| IBIS file stm32u5f9_5g9_ufbga144_dsi_smps.ibs
[IBIS ver] 4.2
[File name] stm32u5f9_5g9_ufbga144_dsi_smps.ibs
[File Rev] 1.0
[Date]  29-10-2024
[Source] Data Created at STMicroelectronics
[Notes]  File originated from ELDO simulations.
[Disclaimer]  This information is for modeling purpose only and is
   not guaranteed. The information is subject to change without
   notice.
[Copyright] Copyright 2024 STMicroelectronics Inc.
|   Component stm32u5f9_5g9_ufbga144_dsi_smps
[Component] stm32u5f9_5g9_ufbga144_dsi_smps
[Manufacturer] STMicroelectronics
[Package]
| variable   typ   min   max
R_pkg  0  NA  NA
L_pkg  0  NA  NA
C_pkg  0  NA  NA
[Pin]   signal_name   model_name
A1  VSS  gnd
A2  PB9  io8_100m_hslv_ft
A3  PH3-BOOT0  io8_100m_ft
A4  PB6  io8_100m_i2c_ft
A5  PB4  io8_100m_hslv_ft
A6  PG14  io8_100m_hslv_ft
A7  PG12  io8_100m_hslv_ft
A8  PG10  io8_100m_hslv_ft
A9  PD7  io8_100m_hslv_ft
A10  PD3  io8_166m_hslv_ft
A11  PC12  io8_166m_hslv_ft
A12  VSS  gnd
B1  PE2  io8_100m_hslv_ft
B2  PE3  io8_100m_hslv_tamp_ft
B3  PE0  io8_100m_hslv_ft
B4  PB8  io8_100m_hslv_ft
B5  PB5  io8_166m_hslv_ft
B6  PG15  io8_100m_hslv_ft
B7  PG9  io8_100m_hslv_ft
B8  PD5  io8_100m_hslv_ft
B9  PD2  io8_100m_hslv_ft
B10  PC10  io8_100m_hslv_ft
B11  PA14  io8_100m_ft
B12  PA10  io8_100m_usb_id
C1  PC14-OSC32_IN   io8_100m_ft
C2  VBAT  power
C3  PE4  io8_100m_hslv_tamp_ft
C4  PE5  io8_100m_hslv_tamp_ft
C5  PB7  io8_166m_hslv_i2c_ft
C6  PG13  io8_100m_hslv_ft
C7  PD4  io8_100m_hslv_ft
C8  PC11  io8_100m_hslv_ft
C9  PA15  nc
C10  PA13  io8_100m_ft
C11  PA12  io8_100m_ft
C12  PA11  io8_100m_ft
D1  VSSDSI  nc
D2  PC15-OSC32_OUT  io8_100m_ft
D3  PE6  io8_100m_hslv_tamp_ft
D4  VDD11  nc
D5  VSS  gnd
D6  PB3  io8_100m_hslv_ft
D7  PD6  io8_166m_hslv_ft
D8  PD0  io8_100m_hslv_ft
D9  VSS  gnd
D10  VDDUSB  power
D11  PA8  io8_166m_hslv_ft
D12  PC8  io8_100m_hslv_ft
E1  DSI_D0N  nc
E2  DSI_D0P  nc
E3  VDDDSI  nc
E4  PC13  io8_100m_ft_v33
E5  PF0  io8_100m_hslv_ft
E6  VDDIO2  power
E7  PD1  io8_100m_hslv_ft
E8  VDD  power
E9  PA9  io8_100m_usb_vbus_ft
E10  VDD  power
E11  PI2  io8_spi_ft
E12  PI3  io8_spi_ft
F1  DSI_CKN  nc
F2  DSI_CKP  nc
F3  VSSDSI  nc
F4  PF1  io8_100m_hslv_ft
F5  VDD  power
F6  VSS  gnd
F7  VSS  gnd
F8  PC9  io8_100m_hslv_ft
F9  PC7  io8_100m_hslv_ft
F10  VSS  gnd
F11  PI0  io8_spi_ft
F12  PI1  io8_spi_ft
G1  DSI_D1N  nc
G2  DSI_D1P  nc
G3  VDD11DSI  nc
G4  PF2  io8_100m_hslv_ft
G5  PC2  io8_100m_hslv_ft
G6  VSS  gnd
G7  VSS  gnd
G8  VDD  power
G9  PC6  io8_100m_hslv_ft
G10  VDD  power
G11  PH14  io8_spi_ft
G12  PH15  io8_spi_ft
H1  VSSDSI  nc
H2  PH0-OSC_IN  io8_100m_ft
H3  VREFP  nc
H4  PA0  io8_100m_hslv_tamp_ft
H5  VDD  power
H6  PB2  io8_100m_hslv_tamp_ft
H7  VDD  power
H8  PE8  io8_100m_hslv_ft
H9  PD15  io8_100m_hslv_ft
H10  VSS  gnd
H11  PH12  io8_spi_ft
H12  PH13  io8_spi_ft
J1  PH1-OSC_OUT  io8_100m_ft
J2  NRST  nc
J3  VSSA  nc
J4  VDDA  nc
J5  PB0  io8_100m_hslv_ft
J6  PG1  io8_100m_hslv_ft
J7  PE10  io8_166m_hslv_ft
J8  PE12  io8_100m_hslv_ft
J9  VDD11  nc
J10  VDD  power
J11  PH11  io8_spi_ft
J12  PH10  io8_spi_ft
K1  PC1  io8_166m_hslv_i2c_ft
K2  PC0  io8_100m_hslv_ft
K3  PA1  io8_100m_hslv_tamp_ft
K4  PA5  io8_100m_ft
K5  PG0  io8_100m_hslv_ft
K6  PE9  io8_166m_hslv_ft
K7  PE14  io8_100m_hslv_ft
K8  PB10  io8_166m_hslv_i2c_ft
K9  PD13  io8_100m_hslv_ft
K10  PD9  io8_100m_hslv_ft
K11  PD12  io8_100m_hslv_ft
K12  PH9  io8_spi_ft
L1  PC3  io8_100m_hslv_ft
L2  PA2  io8_100m_hslv_ft
L3  PA4  io8_100m_hslv_ft
L4  PA7  io8_100m_hslv_ft
L5  PE7  io8_100m_hslv_ft
L6  PE13  io8_100m_hslv_ft
L7  PB11  io8_100m_hslv_ft
L8  VSSSMPS  nc
L9  PD11  io8_100m_hslv_ft
L10  PB14  io8_100m_hslv_ft
L11  PD10  io8_100m_hslv_ft
L12  PD14  io8_100m_hslv_ft
M1  VSS  gnd
M2  PA3  io8_166m_hslv_ft
M3  PA6  io8_100m_hslv_ft
M4  PB1  io8_100m_hslv_ft
M5  PE11  io8_100m_hslv_ft
M6  PE15  io8_100m_hslv_ft
M7  VLXSMPS  nc
M8  VDDSMPS  nc
M9  PB15  nc
M10  PB13  io8_100m_i2c_ft
M11  PD8  io8_100m_hslv_ft
M12  VSS  gnd
[Package Model]   476-ufbga-10x10-144-smps-230223
[Pin Mapping]   pulldown_ref   pullup_ref   | Comment
A1  gndio  nc
A2  gndio  vddiom
A3  gndio  vddiom
A4  gndio  vddiom
A5  gndio  vddiom
A6  gndio  vddiom  | Depending on IO usage
| A6  gndio  vddio2  | Depending on IO usage
A7  gndio  vddiom  | Depending on IO usage
| A7  gndio  vddio2  | Depending on IO usage
A8  gndio  vddiom  | Depending on IO usage
| A8  gndio  vddio2  | Depending on IO usage
A9  gndio  vddiom
A10  gndio  vddiom
A11  gndio  vddiom
A12  gndio  nc
B1  gndio  vddiom
B2  gndio  vddiom
B3  gndio  vddiom
B4  gndio  vddiom
B5  gndio  vddiom
B6  gndio  vddiom  | Depending on IO usage
| B6  gndio  vddio2  | Depending on IO usage
B7  gndio  vddiom  | Depending on IO usage
| B7  gndio  vddio2  | Depending on IO usage
B8  gndio  vddiom
B9  gndio  vddiom
B10  gndio  vddiom
B11  gndio  vddiom
B12  gndio  vddiom  | Depending on IO usage
| B12  gndio  vddusb  | Depending on IO usage
C1  gndio  vddiom  | Depending on IO usage
| C1  gndio  vsw  | Depending on IO usage
C2  nc  vsw
C3  gndio  vddiom
C4  gndio  vddiom
C5  gndio  vddiom
C6  gndio  vddiom  | Depending on IO usage
| C6  gndio  vddio2  | Depending on IO usage
C7  gndio  vddiom
C8  gndio  vddiom
C9  nc  nc
C10  gndio  vddiom  | Depending on IO usage
| C10  gndio  vddusb  | Depending on IO usage
C11  gndio  vddiom  | Depending on IO usage
| C11  gndio  vddusb  | Depending on IO usage
C12  gndio  vddiom  | Depending on IO usage
| C12  gndio  vddusb  | Depending on IO usage
D1  nc  nc
D2  gndio  vddiom  | Depending on IO usage
| D2  gndio  vsw  | Depending on IO usage
D3  gndio  vddiom
D4  nc  nc
D5  gndio  nc
D6  gndio  vddiom
D7  gndio  vddiom
D8  gndio  vddiom
D9  gndio  nc
D10  nc  vddusb
D11  gndio  vddiom
D12  gndio  vddiom
E1  nc  nc
E2  nc  nc
E3  nc  nc
E4  gndio  vddiom  | Depending on IO usage
| E4  gndio  vsw  | Depending on IO usage
E5  gndio  vddiom
E6  nc  vddio2
E7  gndio  vddiom
E8  nc  vddiom
E9  gndio  vddiom  | Depending on IO usage
| E9  gndio  vddusb  | Depending on IO usage
E10  nc  vddhspi
E11  gndio  vddiom  | Depending on IO usage
| E11  gndio  vddhspi  | Depending on IO usage
E12  gndio  vddiom  | Depending on IO usage
| E12  gndio  vddhspi  | Depending on IO usage
F1  nc  nc
F2  nc  nc
F3  nc  nc
F4  gndio  vddiom
F5  nc  vddiom
F6  gndio  nc
F7  gndio  nc
F8  gndio  vddiom
F9  gndio  vddiom
F10  gndio  nc
F11  gndio  vddiom  | Depending on IO usage
| F11  gndio  vddhspi  | Depending on IO usage
F12  gndio  vddiom  | Depending on IO usage
| F12  gndio  vddhspi  | Depending on IO usage
G1  nc  nc
G2  nc  nc
G3  nc  nc
G4  gndio  vddiom
G5  gndio  vddiom
G6  gndio  nc
G7  gndio  nc
G8  nc  vddiom
G9  gndio  vddiom
G10  nc  vddhspi
G11  gndio  vddiom  | Depending on IO usage
| G11  gndio  vddhspi  | Depending on IO usage
G12  gndio  vddiom  | Depending on IO usage
| G12  gndio  vddhspi  | Depending on IO usage
H1  nc  nc
H2  gndio  vddiom
H3  nc  nc
H4  gndio  vddiom
H5  nc  vddiom
H6  gndio  vddiom
H7  nc  vddiom
H8  gndio  vddiom
H9  gndio  vddiom
H10  gndio  nc
H11  gndio  vddiom  | Depending on IO usage
| H11  gndio  vddhspi  | Depending on IO usage
H12  gndio  vddiom  | Depending on IO usage
| H12  gndio  vddhspi  | Depending on IO usage
J1  gndio  vddiom
J2  nc  nc
J3  nc  nc
J4  nc  nc
J5  gndio  vddiom
J6  gndio  vddiom
J7  gndio  vddiom
J8  gndio  vddiom
J9  nc  nc
J10  nc  vddhspi
J11  gndio  vddiom  | Depending on IO usage
| J11  gndio  vddhspi  | Depending on IO usage
J12  gndio  vddiom
K1  gndio  vddiom
K2  gndio  vddiom
K3  gndio  vddiom
K4  gndio  vddiom
K5  gndio  vddiom
K6  gndio  vddiom
K7  gndio  vddiom
K8  gndio  vddiom
K9  gndio  vddiom
K10  gndio  vddiom
K11  gndio  vddiom
K12  gndio  vddiom  | Depending on IO usage
| K12  gndio  vddhspi  | Depending on IO usage
L1  gndio  vddiom
L2  gndio  vddiom
L3  gndio  vddiom
L4  gndio  vddiom
L5  gndio  vddiom
L6  gndio  vddiom
L7  gndio  vddiom
L8  nc  nc
L9  gndio  vddiom
L10  gndio  vddiom
L11  gndio  vddiom
L12  gndio  vddiom
M1  gndio  nc
M2  gndio  vddiom
M3  gndio  vddiom
M4  gndio  vddiom
M5  gndio  vddiom
M6  gndio  vddiom
M7  nc  nc
M8  nc  nc
M9  nc  nc
M10  gndio  vddiom
M11  gndio  vddiom
M12  gndio  nc
[Model Selector] io8_100m_ft
io8_100m_ft_hs_1v2  "IO8_FT 100MHz high speed @ 1.2V"
io8_100m_ft_fs_1v2  "IO8_FT 100MHz fast speed @ 1.2V"
io8_100m_ft_fs_pd_1v2  "IO8_FT 100MHz fast speed @ 1.2V pulldown"
io8_100m_ft_ms_1v2  "IO8_FT 100MHz med speed @ 1.2V"
io8_100m_ft_ms_pd_1v2  "IO8_FT 100MHz med speed @ 1.2V pulldown"
io8_100m_ft_ls_1v2  "IO8_FT 100MHz low speed @ 1.2V"
io8_100m_ft_ls_pd_1v2  "IO8_FT 100MHz low speed @ 1.2V pulldown"
io8_100m_ft_hs_1v8  "IO8_FT 100MHz high speed @ 1.8V"
io8_100m_ft_hs_pd_1v8  "IO8_FT 100MHz high speed @ 1.8V pulldown"
io8_100m_ft_fs_1v8  "IO8_FT 100MHz fast speed @ 1.8V"
io8_100m_ft_fs_pd_1v8  "IO8_FT 100MHz fast speed @ 1.8V pulldown"
io8_100m_ft_ms_1v8  "IO8_FT 100MHz med speed @ 1.8V"
io8_100m_ft_ms_pd_1v8  "IO8_FT 100MHz med speed @ 1.8V pulldown"
io8_100m_ft_ls_1v8  "IO8_FT 100MHz low speed @ 1.8V"
io8_100m_ft_ls_pd_1v8  "IO8_FT 100MHz low speed @ 1.8V pulldown"
io8_100m_ft_hs_3v3  "IO8_FT 100MHz high speed @ 3.3V"
io8_100m_ft_hs_pd_3v3  "IO8_FT 100MHz high speed @ 3.3V pulldown"
io8_100m_ft_fs_3v3  "IO8_FT 100MHz fast speed @ 3.3V"
io8_100m_ft_fs_pd_3v3  "IO8_FT 100MHz fast speed @ 3.3V pulldown"
io8_100m_ft_ms_3v3  "IO8_FT 100MHz med speed @ 3.3V"
io8_100m_ft_ms_pd_3v3  "IO8_FT 100MHz med speed @ 3.3V pulldown"
io8_100m_ft_ls_3v3  "IO8_FT 100MHz low speed @ 3.3V"
io8_100m_ft_ls_pd_3v3  "IO8_FT 100MHz low speed @ 3.3V pulldown"
[Model Selector] io8_100m_hslv_ft
io8_100m_ft_hs_1v2  "IO8_FT 100MHz high speed @ 1.2V"
io8_100m_ft_hs_pu_1v2  "IO8_FT 100MHz high speed @ 1.2V pullup"
io8_100m_ft_hs_pd_1v2  "IO8_FT 100MHz high speed @ 1.2V pulldown"
io8_100m_ft_fs_1v2  "IO8_FT 100MHz fast speed @ 1.2V"
io8_100m_ft_fs_pu_1v2  "IO8_FT 100MHz fast speed @ 1.2V pullup"
io8_100m_ft_fs_pd_1v2  "IO8_FT 100MHz fast speed @ 1.2V pulldown"
io8_100m_ft_ms_1v2  "IO8_FT 100MHz med speed @ 1.2V"
io8_100m_ft_ms_pu_1v2  "IO8_FT 100MHz med speed @ 1.2V pullup"
io8_100m_ft_ms_pd_1v2  "IO8_FT 100MHz med speed @ 1.2V pulldown"
io8_100m_ft_ls_1v2  "IO8_FT 100MHz low speed @ 1.2V"
io8_100m_ft_ls_pu_1v2  "IO8_FT 100MHz low speed @ 1.2V pullup"
io8_100m_ft_ls_pd_1v2  "IO8_FT 100MHz low speed @ 1.2V pulldown"
io8_100m_ft_hs_1v8  "IO8_FT 100MHz high speed @ 1.8V"
io8_100m_ft_hs_pu_1v8  "IO8_FT 100MHz high speed @ 1.8V pullup"
io8_100m_ft_hs_pd_1v8  "IO8_FT 100MHz high speed @ 1.8V pulldown"
io8_100m_ft_fs_1v8  "IO8_FT 100MHz fast speed @ 1.8V"
io8_100m_ft_fs_pu_1v8  "IO8_FT 100MHz fast speed @ 1.8V pullup"
io8_100m_ft_fs_pd_1v8  "IO8_FT 100MHz fast speed @ 1.8V pulldown"
io8_100m_ft_ms_1v8  "IO8_FT 100MHz med speed @ 1.8V"
io8_100m_ft_ms_pu_1v8  "IO8_FT 100MHz med speed @ 1.8V pullup"
io8_100m_ft_ms_pd_1v8  "IO8_FT 100MHz med speed @ 1.8V pulldown"
io8_100m_ft_ls_1v8  "IO8_FT 100MHz low speed @ 1.8V"
io8_100m_ft_ls_pu_1v8  "IO8_FT 100MHz low speed @ 1.8V pullup"
io8_100m_ft_ls_pd_1v8  "IO8_FT 100MHz low speed @ 1.8V pulldown"
io8_100m_ft_hs_3v3  "IO8_FT 100MHz high speed @ 3.3V"
io8_100m_ft_hs_pu_3v3  "IO8_FT 100MHz high speed @ 3.3V pullup"
io8_100m_ft_hs_pd_3v3  "IO8_FT 100MHz high speed @ 3.3V pulldown"
io8_100m_ft_fs_3v3  "IO8_FT 100MHz fast speed @ 3.3V"
io8_100m_ft_fs_pu_3v3  "IO8_FT 100MHz fast speed @ 3.3V pullup"
io8_100m_ft_fs_pd_3v3  "IO8_FT 100MHz fast speed @ 3.3V pulldown"
io8_100m_ft_ms_3v3  "IO8_FT 100MHz med speed @ 3.3V"
io8_100m_ft_ms_pu_3v3  "IO8_FT 100MHz med speed @ 3.3V pullup"
io8_100m_ft_ms_pd_3v3  "IO8_FT 100MHz med speed @ 3.3V pulldown"
io8_100m_ft_ls_3v3  "IO8_FT 100MHz low speed @ 3.3V"
io8_100m_ft_ls_pu_3v3  "IO8_FT 100MHz low speed @ 3.3V pullup"
io8_100m_ft_ls_pd_3v3  "IO8_FT 100MHz low speed @ 3.3V pulldown"
io8_100m_hslv_ft_hs_1v2  "IO8_FT 100MHz HSLV high speed @ 1.2V"
io8_100m_hslv_ft_hs_pu_1v2  "IO8_FT 100MHz HSLV high speed @ 1.2V pullup"
io8_100m_hslv_ft_hs_pd_1v2  "IO8_FT 100MHz HSLV high speed @ 1.2V pulldown"
io8_100m_hslv_ft_fs_1v2  "IO8_FT 100MHz HSLV fast speed @ 1.2V"
io8_100m_hslv_ft_fs_pu_1v2  "IO8_FT 100MHz HSLV fast speed @ 1.2V pullup"
io8_100m_hslv_ft_fs_pd_1v2  "IO8_FT 100MHz HSLV fast speed @ 1.2V pulldown"
io8_100m_hslv_ft_ms_1v2  "IO8_FT 100MHz HSLV med speed @ 1.2V"
io8_100m_hslv_ft_ms_pu_1v2  "IO8_FT 100MHz HSLV med speed @ 1.2V pullup"
io8_100m_hslv_ft_ms_pd_1v2  "IO8_FT 100MHz HSLV med speed @ 1.2V pulldown"
io8_100m_hslv_ft_ls_1v2  "IO8_FT 100MHz HSLV low speed @ 1.2V"
io8_100m_hslv_ft_ls_pu_1v2  "IO8_FT 100MHz HSLV low speed @ 1.2V pullup"
io8_100m_hslv_ft_ls_pd_1v2  "IO8_FT 100MHz HSLV low speed @ 1.2V pulldown"
io8_100m_hslv_ft_hs_1v8  "IO8_FT 100MHz HSLV high speed @ 1.8V"
io8_100m_hslv_ft_hs_pu_1v8  "IO8_FT 100MHz HSLV high speed @ 1.8V pullup"
io8_100m_hslv_ft_hs_pd_1v8  "IO8_FT 100MHz HSLV high speed @ 1.8V pulldown"
io8_100m_hslv_ft_fs_1v8  "IO8_FT 100MHz HSLV fast speed @ 1.8V"
io8_100m_hslv_ft_fs_pu_1v8  "IO8_FT 100MHz HSLV fast speed @ 1.8V pullup"
io8_100m_hslv_ft_fs_pd_1v8  "IO8_FT 100MHz HSLV fast speed @ 1.8V pulldown"
io8_100m_hslv_ft_ms_1v8  "IO8_FT 100MHz HSLV med speed @ 1.8V"
io8_100m_hslv_ft_ms_pu_1v8  "IO8_FT 100MHz HSLV med speed @ 1.8V pullup"
io8_100m_hslv_ft_ms_pd_1v8  "IO8_FT 100MHz HSLV med speed @ 1.8V pulldown"
io8_100m_hslv_ft_ls_1v8  "IO8_FT 100MHz HSLV low speed @ 1.8V"
io8_100m_hslv_ft_ls_pu_1v8  "IO8_FT 100MHz HSLV low speed @ 1.8V pullup"
io8_100m_hslv_ft_ls_pd_1v8  "IO8_FT 100MHz HSLV low speed @ 1.8V pulldown"
io8_100m_hslv_ft_hs_2v5  "IO8_FT 100MHz HSLV high speed @ 2.5V"
io8_100m_hslv_ft_hs_pu_2v5  "IO8_FT 100MHz HSLV high speed @ 2.5V pullup"
io8_100m_hslv_ft_hs_pd_2v5  "IO8_FT 100MHz HSLV high speed @ 2.5V pulldown"
io8_100m_hslv_ft_fs_2v5  "IO8_FT 100MHz HSLV fast speed @ 2.5V"
io8_100m_hslv_ft_fs_pu_2v5  "IO8_FT 100MHz HSLV fast speed @ 2.5V pullup"
io8_100m_hslv_ft_fs_pd_2v5  "IO8_FT 100MHz HSLV fast speed @ 2.5V pulldown"
io8_100m_hslv_ft_ms_2v5  "IO8_FT 100MHz HSLV med speed @ 2.5V"
io8_100m_hslv_ft_ms_pu_2v5  "IO8_FT 100MHz HSLV med speed @ 2.5V pullup"
io8_100m_hslv_ft_ms_pd_2v5  "IO8_FT 100MHz HSLV med speed @ 2.5V pulldown"
io8_100m_hslv_ft_ls_2v5  "IO8_FT 100MHz HSLV low speed @ 2.5V"
io8_100m_hslv_ft_ls_pu_2v5  "IO8_FT 100MHz HSLV low speed @ 2.5V pullup"
io8_100m_hslv_ft_ls_pd_2v5  "IO8_FT 100MHz HSLV low speed @ 2.5V pulldown"
[Model Selector] io8_100m_hslv_tamp_ft
io8_100m_ft_hs_1v2  "IO8_FT 100MHz high speed @ 1.2V"
io8_100m_ft_hs_pu_1v2  "IO8_FT 100MHz high speed @ 1.2V pullup"
io8_100m_ft_hs_pd_1v2  "IO8_FT 100MHz high speed @ 1.2V pulldown"
io8_100m_ft_fs_1v2  "IO8_FT 100MHz fast speed @ 1.2V"
io8_100m_ft_fs_pu_1v2  "IO8_FT 100MHz fast speed @ 1.2V pullup"
io8_100m_ft_fs_pd_1v2  "IO8_FT 100MHz fast speed @ 1.2V pulldown"
io8_100m_ft_ms_1v2  "IO8_FT 100MHz med speed @ 1.2V"
io8_100m_ft_ms_pu_1v2  "IO8_FT 100MHz med speed @ 1.2V pullup"
io8_100m_ft_ms_pd_1v2  "IO8_FT 100MHz med speed @ 1.2V pulldown"
io8_100m_ft_ls_1v2  "IO8_FT 100MHz low speed @ 1.2V"
io8_100m_ft_ls_pu_1v2  "IO8_FT 100MHz low speed @ 1.2V pullup"
io8_100m_ft_ls_pd_1v2  "IO8_FT 100MHz low speed @ 1.2V pulldown"
io8_100m_ft_hs_1v8  "IO8_FT 100MHz high speed @ 1.8V"
io8_100m_ft_hs_pu_1v8  "IO8_FT 100MHz high speed @ 1.8V pullup"
io8_100m_ft_hs_pd_1v8  "IO8_FT 100MHz high speed @ 1.8V pulldown"
io8_100m_ft_fs_1v8  "IO8_FT 100MHz fast speed @ 1.8V"
io8_100m_ft_fs_pu_1v8  "IO8_FT 100MHz fast speed @ 1.8V pullup"
io8_100m_ft_fs_pd_1v8  "IO8_FT 100MHz fast speed @ 1.8V pulldown"
io8_100m_ft_ms_1v8  "IO8_FT 100MHz med speed @ 1.8V"
io8_100m_ft_ms_pu_1v8  "IO8_FT 100MHz med speed @ 1.8V pullup"
io8_100m_ft_ms_pd_1v8  "IO8_FT 100MHz med speed @ 1.8V pulldown"
io8_100m_ft_ls_1v8  "IO8_FT 100MHz low speed @ 1.8V"
io8_100m_ft_ls_pu_1v8  "IO8_FT 100MHz low speed @ 1.8V pullup"
io8_100m_ft_ls_pd_1v8  "IO8_FT 100MHz low speed @ 1.8V pulldown"
io8_100m_ft_hs_3v3  "IO8_FT 100MHz high speed @ 3.3V"
io8_100m_ft_hs_pu_3v3  "IO8_FT 100MHz high speed @ 3.3V pullup"
io8_100m_ft_hs_pd_3v3  "IO8_FT 100MHz high speed @ 3.3V pulldown"
io8_100m_ft_fs_3v3  "IO8_FT 100MHz fast speed @ 3.3V"
io8_100m_ft_fs_pu_3v3  "IO8_FT 100MHz fast speed @ 3.3V pullup"
io8_100m_ft_fs_pd_3v3  "IO8_FT 100MHz fast speed @ 3.3V pulldown"
io8_100m_ft_ms_3v3  "IO8_FT 100MHz med speed @ 3.3V"
io8_100m_ft_ms_pu_3v3  "IO8_FT 100MHz med speed @ 3.3V pullup"
io8_100m_ft_ms_pd_3v3  "IO8_FT 100MHz med speed @ 3.3V pulldown"
io8_100m_ft_ls_3v3  "IO8_FT 100MHz low speed @ 3.3V"
io8_100m_ft_ls_pu_3v3  "IO8_FT 100MHz low speed @ 3.3V pullup"
io8_100m_ft_ls_pd_3v3  "IO8_FT 100MHz low speed @ 3.3V pulldown"
io8_100m_hslv_ft_hs_1v2  "IO8_FT 100MHz HSLV high speed @ 1.2V"
io8_100m_hslv_ft_hs_pu_1v2  "IO8_FT 100MHz HSLV high speed @ 1.2V pullup"
io8_100m_hslv_ft_hs_pd_1v2  "IO8_FT 100MHz HSLV high speed @ 1.2V pulldown"
io8_100m_hslv_ft_fs_1v2  "IO8_FT 100MHz HSLV fast speed @ 1.2V"
io8_100m_hslv_ft_fs_pu_1v2  "IO8_FT 100MHz HSLV fast speed @ 1.2V pullup"
io8_100m_hslv_ft_fs_pd_1v2  "IO8_FT 100MHz HSLV fast speed @ 1.2V pulldown"
io8_100m_hslv_ft_ms_1v2  "IO8_FT 100MHz HSLV med speed @ 1.2V"
io8_100m_hslv_ft_ms_pu_1v2  "IO8_FT 100MHz HSLV med speed @ 1.2V pullup"
io8_100m_hslv_ft_ms_pd_1v2  "IO8_FT 100MHz HSLV med speed @ 1.2V pulldown"
io8_100m_hslv_ft_ls_1v2  "IO8_FT 100MHz HSLV low speed @ 1.2V"
io8_100m_hslv_ft_ls_pu_1v2  "IO8_FT 100MHz HSLV low speed @ 1.2V pullup"
io8_100m_hslv_ft_ls_pd_1v2  "IO8_FT 100MHz HSLV low speed @ 1.2V pulldown"
io8_100m_hslv_ft_hs_1v8  "IO8_FT 100MHz HSLV high speed @ 1.8V"
io8_100m_hslv_ft_hs_pu_1v8  "IO8_FT 100MHz HSLV high speed @ 1.8V pullup"
io8_100m_hslv_ft_hs_pd_1v8  "IO8_FT 100MHz HSLV high speed @ 1.8V pulldown"
io8_100m_hslv_ft_fs_1v8  "IO8_FT 100MHz HSLV fast speed @ 1.8V"
io8_100m_hslv_ft_fs_pu_1v8  "IO8_FT 100MHz HSLV fast speed @ 1.8V pullup"
io8_100m_hslv_ft_fs_pd_1v8  "IO8_FT 100MHz HSLV fast speed @ 1.8V pulldown"
io8_100m_hslv_ft_ms_1v8  "IO8_FT 100MHz HSLV med speed @ 1.8V"
io8_100m_hslv_ft_ms_pu_1v8  "IO8_FT 100MHz HSLV med speed @ 1.8V pullup"
io8_100m_hslv_ft_ms_pd_1v8  "IO8_FT 100MHz HSLV med speed @ 1.8V pulldown"
io8_100m_hslv_ft_ls_1v8  "IO8_FT 100MHz HSLV low speed @ 1.8V"
io8_100m_hslv_ft_ls_pu_1v8  "IO8_FT 100MHz HSLV low speed @ 1.8V pullup"
io8_100m_hslv_ft_ls_pd_1v8  "IO8_FT 100MHz HSLV low speed @ 1.8V pulldown"
io8_100m_hslv_ft_hs_2v5  "IO8_FT 100MHz HSLV high speed @ 2.5V"
io8_100m_hslv_ft_hs_pu_2v5  "IO8_FT 100MHz HSLV high speed @ 2.5V pullup"
io8_100m_hslv_ft_hs_pd_2v5  "IO8_FT 100MHz HSLV high speed @ 2.5V pulldown"
io8_100m_hslv_ft_fs_2v5  "IO8_FT 100MHz HSLV fast speed @ 2.5V"
io8_100m_hslv_ft_fs_pu_2v5  "IO8_FT 100MHz HSLV fast speed @ 2.5V pullup"
io8_100m_hslv_ft_fs_pd_2v5  "IO8_FT 100MHz HSLV fast speed @ 2.5V pulldown"
io8_100m_hslv_ft_ms_2v5  "IO8_FT 100MHz HSLV med speed @ 2.5V"
io8_100m_hslv_ft_ms_pu_2v5  "IO8_FT 100MHz HSLV med speed @ 2.5V pullup"
io8_100m_hslv_ft_ms_pd_2v5  "IO8_FT 100MHz HSLV med speed @ 2.5V pulldown"
io8_100m_hslv_ft_ls_2v5  "IO8_FT 100MHz HSLV low speed @ 2.5V"
io8_100m_hslv_ft_ls_pu_2v5  "IO8_FT 100MHz HSLV low speed @ 2.5V pullup"
io8_100m_hslv_ft_ls_pd_2v5  "IO8_FT 100MHz HSLV low speed @ 2.5V pulldown"
io8_ft_v33_hs_1v2  "IO8_FT_V33 high speed @ 1.2V"
io8_ft_v33_hs_pu_1v2  "IO8_FT_V33 high speed @ 1.2V pullup"
io8_ft_v33_hs_pd_1v2  "IO8_FT_V33 high speed @ 1.2V pulldown"
io8_ft_v33_fs_1v2  "IO8_FT_V33 fast speed @ 1.2V"
io8_ft_v33_fs_pu_1v2  "IO8_FT_V33 fast speed @ 1.2V pullup"
io8_ft_v33_fs_pd_1v2  "IO8_FT_V33 fast speed @ 1.2V pulldown"
io8_ft_v33_ms_1v2  "IO8_FT_V33 med speed @ 1.2V"
io8_ft_v33_ms_pu_1v2  "IO8_FT_V33 med speed @ 1.2V pullup"
io8_ft_v33_ms_pd_1v2  "IO8_FT_V33 med speed @ 1.2V pulldown"
io8_ft_v33_ls_1v2  "IO8_FT_V33 low speed @ 1.2V"
io8_ft_v33_ls_pu_1v2  "IO8_FT_V33 low speed @ 1.2V pullup"
io8_ft_v33_ls_pd_1v2  "IO8_FT_V33 low speed @ 1.2V pulldown"
io8_ft_v33_hs_1v8  "IO8_FT_V33 high speed @ 1.8V"
io8_ft_v33_hs_pu_1v8  "IO8_FT_V33 high speed @ 1.8V pullup"
io8_ft_v33_hs_pd_1v8  "IO8_FT_V33 high speed @ 1.8V pulldown"
io8_ft_v33_fs_1v8  "IO8_FT_V33 fast speed @ 1.8V"
io8_ft_v33_fs_pu_1v8  "IO8_FT_V33 fast speed @ 1.8V pullup"
io8_ft_v33_fs_pd_1v8  "IO8_FT_V33 fast speed @ 1.8V pulldown"
io8_ft_v33_ms_1v8  "IO8_FT_V33 med speed @ 1.8V"
io8_ft_v33_ms_pu_1v8  "IO8_FT_V33 med speed @ 1.8V pullup"
io8_ft_v33_ms_pd_1v8  "IO8_FT_V33 med speed @ 1.8V pulldown"
io8_ft_v33_ls_1v8  "IO8_FT_V33 low speed @ 1.8V"
io8_ft_v33_ls_pu_1v8  "IO8_FT_V33 low speed @ 1.8V pullup"
io8_ft_v33_ls_pd_1v8  "IO8_FT_V33 low speed @ 1.8V pulldown"
io8_ft_v33_hs_3v3  "IO8_FT_V33 high speed @ 3.3V"
io8_ft_v33_hs_pu_3v3  "IO8_FT_V33 high speed @ 3.3V pullup"
io8_ft_v33_hs_pd_3v3  "IO8_FT_V33 high speed @ 3.3V pulldown"
io8_ft_v33_fs_3v3  "IO8_FT_V33 fast speed @ 3.3V"
io8_ft_v33_fs_pu_3v3  "IO8_FT_V33 fast speed @ 3.3V pullup"
io8_ft_v33_fs_pd_3v3  "IO8_FT_V33 fast speed @ 3.3V pulldown"
io8_ft_v33_ms_3v3  "IO8_FT_V33 med speed @ 3.3V"
io8_ft_v33_ms_pu_3v3  "IO8_FT_V33 med speed @ 3.3V pullup"
io8_ft_v33_ms_pd_3v3  "IO8_FT_V33 med speed @ 3.3V pulldown"
io8_ft_v33_ls_3v3  "IO8_FT_V33 low speed @ 3.3V"
io8_ft_v33_ls_pu_3v3  "IO8_FT_V33 low speed @ 3.3V pullup"
io8_ft_v33_ls_pd_3v3  "IO8_FT_V33 low speed @ 3.3V pulldown"
[Model Selector] io8_100m_i2c_ft
io8_100m_ft_hs_1v2  "IO8_FT 100MHz high speed @ 1.2V"
io8_100m_ft_hs_pu_1v2  "IO8_FT 100MHz high speed @ 1.2V pullup"
io8_100m_ft_hs_pd_1v2  "IO8_FT 100MHz high speed @ 1.2V pulldown"
io8_100m_ft_fs_1v2  "IO8_FT 100MHz fast speed @ 1.2V"
io8_100m_ft_fs_pu_1v2  "IO8_FT 100MHz fast speed @ 1.2V pullup"
io8_100m_ft_fs_pd_1v2  "IO8_FT 100MHz fast speed @ 1.2V pulldown"
io8_100m_ft_ms_1v2  "IO8_FT 100MHz med speed @ 1.2V"
io8_100m_ft_ms_pu_1v2  "IO8_FT 100MHz med speed @ 1.2V pullup"
io8_100m_ft_ms_pd_1v2  "IO8_FT 100MHz med speed @ 1.2V pulldown"
io8_100m_ft_ls_1v2  "IO8_FT 100MHz low speed @ 1.2V"
io8_100m_ft_ls_pu_1v2  "IO8_FT 100MHz low speed @ 1.2V pullup"
io8_100m_ft_ls_pd_1v2  "IO8_FT 100MHz low speed @ 1.2V pulldown"
io8_100m_ft_hs_1v8  "IO8_FT 100MHz high speed @ 1.8V"
io8_100m_ft_hs_pu_1v8  "IO8_FT 100MHz high speed @ 1.8V pullup"
io8_100m_ft_hs_pd_1v8  "IO8_FT 100MHz high speed @ 1.8V pulldown"
io8_100m_ft_fs_1v8  "IO8_FT 100MHz fast speed @ 1.8V"
io8_100m_ft_fs_pu_1v8  "IO8_FT 100MHz fast speed @ 1.8V pullup"
io8_100m_ft_fs_pd_1v8  "IO8_FT 100MHz fast speed @ 1.8V pulldown"
io8_100m_ft_ms_1v8  "IO8_FT 100MHz med speed @ 1.8V"
io8_100m_ft_ms_pu_1v8  "IO8_FT 100MHz med speed @ 1.8V pullup"
io8_100m_ft_ms_pd_1v8  "IO8_FT 100MHz med speed @ 1.8V pulldown"
io8_100m_ft_ls_1v8  "IO8_FT 100MHz low speed @ 1.8V"
io8_100m_ft_ls_pu_1v8  "IO8_FT 100MHz low speed @ 1.8V pullup"
io8_100m_ft_ls_pd_1v8  "IO8_FT 100MHz low speed @ 1.8V pulldown"
io8_100m_ft_hs_3v3  "IO8_FT 100MHz high speed @ 3.3V"
io8_100m_ft_hs_pu_3v3  "IO8_FT 100MHz high speed @ 3.3V pullup"
io8_100m_ft_hs_pd_3v3  "IO8_FT 100MHz high speed @ 3.3V pulldown"
io8_100m_ft_fs_3v3  "IO8_FT 100MHz fast speed @ 3.3V"
io8_100m_ft_fs_pu_3v3  "IO8_FT 100MHz fast speed @ 3.3V pullup"
io8_100m_ft_fs_pd_3v3  "IO8_FT 100MHz fast speed @ 3.3V pulldown"
io8_100m_ft_ms_3v3  "IO8_FT 100MHz med speed @ 3.3V"
io8_100m_ft_ms_pu_3v3  "IO8_FT 100MHz med speed @ 3.3V pullup"
io8_100m_ft_ms_pd_3v3  "IO8_FT 100MHz med speed @ 3.3V pulldown"
io8_100m_ft_ls_3v3  "IO8_FT 100MHz low speed @ 3.3V"
io8_100m_ft_ls_pu_3v3  "IO8_FT 100MHz low speed @ 3.3V pullup"
io8_100m_ft_ls_pd_3v3  "IO8_FT 100MHz low speed @ 3.3V pulldown"
io8_100m_i2c_ft_1v2  "IO8_FT 100MHz I2C @ 1.2V"
io8_100m_i2c_ft_pu_1v2  "IO8_FT 100MHz I2C @ 1.2V pullup"
io8_100m_i2c_ft_pd_1v2  "IO8_FT 100MHz I2C @ 1.2V pulldown"
io8_100m_i2c_ft_1v8  "IO8_FT 100MHz I2C @ 1.8V"
io8_100m_i2c_ft_pu_1v8  "IO8_FT 100MHz I2C @ 1.8V pullup"
io8_100m_i2c_ft_pd_1v8  "IO8_FT 100MHz I2C @ 1,8V pulldown"
io8_100m_i2c_ft_3v3  "IO8_FT 100MHz I2C @ 3.3V"
io8_100m_i2c_ft_pu_3v3  "IO8_FT 100MHz I2C HSLV @ 3.3V pullup"
io8_100m_i2c_ft_pd_3v3  "IO8_FT 100MHz I2C @ 3.3V pulldown"
[Model Selector] io8_100m_usb_id
io8_100m_ft_hs_1v2  "IO8_FT 100MHz high speed @ 1.2V"
io8_100m_ft_hs_pu_1v2  "IO8_FT 100MHz high speed @ 1.2V pullup"
io8_100m_ft_hs_pd_1v2  "IO8_FT 100MHz high speed @ 1.2V pulldown"
io8_100m_ft_fs_1v2  "IO8_FT 100MHz fast speed @ 1.2V"
io8_100m_ft_fs_pu_1v2  "IO8_FT 100MHz fast speed @ 1.2V pullup"
io8_100m_ft_fs_pd_1v2  "IO8_FT 100MHz fast speed @ 1.2V pulldown"
io8_100m_ft_ms_1v2  "IO8_FT 100MHz med speed @ 1.2V"
io8_100m_ft_ms_pu_1v2  "IO8_FT 100MHz med speed @ 1.2V pullup"
io8_100m_ft_ms_pd_1v2  "IO8_FT 100MHz med speed @ 1.2V pulldown"
io8_100m_ft_ls_1v2  "IO8_FT 100MHz low speed @ 1.2V"
io8_100m_ft_ls_pu_1v2  "IO8_FT 100MHz low speed @ 1.2V pullup"
io8_100m_ft_ls_pd_1v2  "IO8_FT 100MHz low speed @ 1.2V pulldown"
io8_100m_ft_hs_1v8  "IO8_FT 100MHz high speed @ 1.8V"
io8_100m_ft_hs_pu_1v8  "IO8_FT 100MHz high speed @ 1.8V pullup"
io8_100m_ft_hs_pd_1v8  "IO8_FT 100MHz high speed @ 1.8V pulldown"
io8_100m_ft_fs_1v8  "IO8_FT 100MHz fast speed @ 1.8V"
io8_100m_ft_fs_pu_1v8  "IO8_FT 100MHz fast speed @ 1.8V pullup"
io8_100m_ft_fs_pd_1v8  "IO8_FT 100MHz fast speed @ 1.8V pulldown"
io8_100m_ft_ms_1v8  "IO8_FT 100MHz med speed @ 1.8V"
io8_100m_ft_ms_pu_1v8  "IO8_FT 100MHz med speed @ 1.8V pullup"
io8_100m_ft_ms_pd_1v8  "IO8_FT 100MHz med speed @ 1.8V pulldown"
io8_100m_ft_ls_1v8  "IO8_FT 100MHz low speed @ 1.8V"
io8_100m_ft_ls_pu_1v8  "IO8_FT 100MHz low speed @ 1.8V pullup"
io8_100m_ft_ls_pd_1v8  "IO8_FT 100MHz low speed @ 1.8V pulldown"
io8_100m_ft_hs_3v3  "IO8_FT 100MHz high speed @ 3.3V"
io8_100m_ft_hs_pu_3v3  "IO8_FT 100MHz high speed @ 3.3V pullup"
io8_100m_ft_hs_pd_3v3  "IO8_FT 100MHz high speed @ 3.3V pulldown"
io8_100m_ft_fs_3v3  "IO8_FT 100MHz fast speed @ 3.3V"
io8_100m_ft_fs_pu_3v3  "IO8_FT 100MHz fast speed @ 3.3V pullup"
io8_100m_ft_fs_pd_3v3  "IO8_FT 100MHz fast speed @ 3.3V pulldown"
io8_100m_ft_ms_3v3  "IO8_FT 100MHz med speed @ 3.3V"
io8_100m_ft_ms_pu_3v3  "IO8_FT 100MHz med speed @ 3.3V pullup"
io8_100m_ft_ms_pd_3v3  "IO8_FT 100MHz med speed @ 3.3V pulldown"
io8_100m_ft_ls_3v3  "IO8_FT 100MHz low speed @ 3.3V"
io8_100m_ft_ls_pu_3v3  "IO8_FT 100MHz low speed @ 3.3V pullup"
io8_100m_ft_ls_pd_3v3  "IO8_FT 100MHz low speed @ 3.3V pulldown"
io8usb_id_nopu  "IOUSB ID @ 3.3V"
io8usb_id_pu  "IOUSB ID @ 3.3V pullup"
[Model Selector] io8_100m_usb_vbus_ft
io8_100m_ft_hs_1v2  "IO8_FT 100MHz high speed @ 1.2V"
io8_100m_ft_hs_pu_1v2  "IO8_FT 100MHz high speed @ 1.2V pullup"
io8_100m_ft_hs_pd_1v2  "IO8_FT 100MHz high speed @ 1.2V pulldown"
io8_100m_ft_fs_1v2  "IO8_FT 100MHz fast speed @ 1.2V"
io8_100m_ft_fs_pu_1v2  "IO8_FT 100MHz fast speed @ 1.2V pullup"
io8_100m_ft_fs_pd_1v2  "IO8_FT 100MHz fast speed @ 1.2V pulldown"
io8_100m_ft_ms_1v2  "IO8_FT 100MHz med speed @ 1.2V"
io8_100m_ft_ms_pu_1v2  "IO8_FT 100MHz med speed @ 1.2V pullup"
io8_100m_ft_ms_pd_1v2  "IO8_FT 100MHz med speed @ 1.2V pulldown"
io8_100m_ft_ls_1v2  "IO8_FT 100MHz low speed @ 1.2V"
io8_100m_ft_ls_pu_1v2  "IO8_FT 100MHz low speed @ 1.2V pullup"
io8_100m_ft_ls_pd_1v2  "IO8_FT 100MHz low speed @ 1.2V pulldown"
io8_100m_ft_hs_1v8  "IO8_FT 100MHz high speed @ 1.8V"
io8_100m_ft_hs_pu_1v8  "IO8_FT 100MHz high speed @ 1.8V pullup"
io8_100m_ft_hs_pd_1v8  "IO8_FT 100MHz high speed @ 1.8V pulldown"
io8_100m_ft_fs_1v8  "IO8_FT 100MHz fast speed @ 1.8V"
io8_100m_ft_fs_pu_1v8  "IO8_FT 100MHz fast speed @ 1.8V pullup"
io8_100m_ft_fs_pd_1v8  "IO8_FT 100MHz fast speed @ 1.8V pulldown"
io8_100m_ft_ms_1v8  "IO8_FT 100MHz med speed @ 1.8V"
io8_100m_ft_ms_pu_1v8  "IO8_FT 100MHz med speed @ 1.8V pullup"
io8_100m_ft_ms_pd_1v8  "IO8_FT 100MHz med speed @ 1.8V pulldown"
io8_100m_ft_ls_1v8  "IO8_FT 100MHz low speed @ 1.8V"
io8_100m_ft_ls_pu_1v8  "IO8_FT 100MHz low speed @ 1.8V pullup"
io8_100m_ft_ls_pd_1v8  "IO8_FT 100MHz low speed @ 1.8V pulldown"
io8_100m_ft_hs_3v3  "IO8_FT 100MHz high speed @ 3.3V"
io8_100m_ft_hs_pu_3v3  "IO8_FT 100MHz high speed @ 3.3V pullup"
io8_100m_ft_hs_pd_3v3  "IO8_FT 100MHz high speed @ 3.3V pulldown"
io8_100m_ft_fs_3v3  "IO8_FT 100MHz fast speed @ 3.3V"
io8_100m_ft_fs_pu_3v3  "IO8_FT 100MHz fast speed @ 3.3V pullup"
io8_100m_ft_fs_pd_3v3  "IO8_FT 100MHz fast speed @ 3.3V pulldown"
io8_100m_ft_ms_3v3  "IO8_FT 100MHz med speed @ 3.3V"
io8_100m_ft_ms_pu_3v3  "IO8_FT 100MHz med speed @ 3.3V pullup"
io8_100m_ft_ms_pd_3v3  "IO8_FT 100MHz med speed @ 3.3V pulldown"
io8_100m_ft_ls_3v3  "IO8_FT 100MHz low speed @ 3.3V"
io8_100m_ft_ls_pu_3v3  "IO8_FT 100MHz low speed @ 3.3V pullup"
io8_100m_ft_ls_pd_3v3  "IO8_FT 100MHz low speed @ 3.3V pulldown"
io8usb_adp "IOUSB ADP @ 3.3V"
io8usb_vbus "IOUSB VBUS @ 3.3V"
[Model Selector] io8_166m_hslv_ft
io8_166m_ft_hs_1v2  "IO8_FT 166MHz high speed @ 1.2V"
io8_166m_ft_hs_pu_1v2  "IO8_FT 166MHz high speed @ 1.2V pullup"
io8_166m_ft_hs_pd_1v2  "IO8_FT 166MHz high speed @ 1.2V pulldown"
io8_166m_ft_fs_1v2  "IO8_FT 166MHz fast speed @ 1.2V"
io8_166m_ft_fs_pu_1v2  "IO8_FT 166MHz fast speed @ 1.2V pullup"
io8_166m_ft_fs_pd_1v2  "IO8_FT 166MHz fast speed @ 1.2V pulldown"
io8_166m_ft_ms_1v2  "IO8_FT 166MHz med speed @ 1.2V"
io8_166m_ft_ms_pu_1v2  "IO8_FT 166MHz med speed @ 1.2V pullup"
io8_166m_ft_ms_pd_1v2  "IO8_FT 166MHz med speed @ 1.2V pulldown"
io8_166m_ft_ls_1v2  "IO8_FT 166MHz low speed @ 1.2V"
io8_166m_ft_ls_pu_1v2  "IO8_FT 166MHz low speed @ 1.2V pullup"
io8_166m_ft_ls_pd_1v2  "IO8_FT 166MHz low speed @ 1.2V pulldown"
io8_166m_ft_hs_1v8  "IO8_FT 166MHz high speed @ 1.8V"
io8_166m_ft_hs_pu_1v8  "IO8_FT 166MHz high speed @ 1.8V pullup"
io8_166m_ft_hs_pd_1v8  "IO8_FT 166MHz high speed @ 1.8V pulldown"
io8_166m_ft_fs_1v8  "IO8_FT 166MHz fast speed @ 1.8V"
io8_166m_ft_fs_pu_1v8  "IO8_FT 166MHz fast speed @ 1.8V pullup"
io8_166m_ft_fs_pd_1v8  "IO8_FT 166MHz fast speed @ 1.8V pulldown"
io8_166m_ft_ms_1v8  "IO8_FT 166MHz med speed @ 1.8V"
io8_166m_ft_ms_pu_1v8  "IO8_FT 166MHz med speed @ 1.8V pullup"
io8_166m_ft_ms_pd_1v8  "IO8_FT 166MHz med speed @ 1.8V pulldown"
io8_166m_ft_ls_1v8  "IO8_FT 166MHz low speed @ 1.8V"
io8_166m_ft_ls_pu_1v8  "IO8_FT 166MHz low speed @ 1.8V pullup"
io8_166m_ft_ls_pd_1v8  "IO8_FT 166MHz low speed @ 1.8V pulldown"
io8_166m_ft_hs_3v3  "IO8_FT 166MHz high speed @ 3.3V"
io8_166m_ft_hs_pu_3v3  "IO8_FT 166MHz high speed @ 3.3V pullup"
io8_166m_ft_hs_pd_3v3  "IO8_FT 166MHz high speed @ 3.3V pulldown"
io8_166m_ft_fs_3v3  "IO8_FT 166MHz fast speed @ 3.3V"
io8_166m_ft_fs_pu_3v3  "IO8_FT 166MHz fast speed @ 3.3V pullup"
io8_166m_ft_fs_pd_3v3  "IO8_FT 166MHz fast speed @ 3.3V pulldown"
io8_166m_ft_ms_3v3  "IO8_FT 166MHz med speed @ 3.3V"
io8_166m_ft_ms_pu_3v3  "IO8_FT 166MHz med speed @ 3.3V pullup"
io8_166m_ft_ms_pd_3v3  "IO8_FT 166MHz med speed @ 3.3V pulldown"
io8_166m_ft_ls_3v3  "IO8_FT 166MHz low speed @ 3.3V"
io8_166m_ft_ls_pu_3v3  "IO8_FT 166MHz low speed @ 3.3V pullup"
io8_166m_ft_ls_pd_3v3  "IO8_FT 166MHz low speed @ 3.3V pulldown"
io8_166m_hslv_ft_hs_1v2  "IO8_FT 166MHz HSLV high speed @ 1.2V"
io8_166m_hslv_ft_hs_pu_1v2  "IO8_FT 166MHz HSLV high speed @ 1.2V pullup"
io8_166m_hslv_ft_hs_pd_1v2  "IO8_FT 166MHz HSLV high speed @ 1.2V pulldown"
io8_166m_hslv_ft_fs_1v2  "IO8_FT 166MHz HSLV fast speed @ 1.2V"
io8_166m_hslv_ft_fs_pu_1v2  "IO8_FT 166MHz HSLV fast speed @ 1.2V pullup"
io8_166m_hslv_ft_fs_pd_1v2  "IO8_FT 166MHz HSLV fast speed @ 1.2V pulldown"
io8_166m_hslv_ft_ms_1v2  "IO8_FT 166MHz HSLV med speed @ 1.2V"
io8_166m_hslv_ft_ms_pu_1v2  "IO8_FT 166MHz HSLV med speed @ 1.2V pullup"
io8_166m_hslv_ft_ms_pd_1v2  "IO8_FT 166MHz HSLV med speed @ 1.2V pulldown"
io8_166m_hslv_ft_ls_1v2  "IO8_FT 166MHz HSLV low speed @ 1.2V"
io8_166m_hslv_ft_ls_pu_1v2  "IO8_FT 166MHz HSLV low speed @ 1.2V pullup"
io8_166m_hslv_ft_ls_pd_1v2  "IO8_FT 166MHz HSLV low speed @ 1.2V pulldown"
io8_166m_hslv_ft_hs_1v8  "IO8_FT 166MHz HSLV high speed @ 1.8V"
io8_166m_hslv_ft_hs_pu_1v8  "IO8_FT 166MHz HSLV high speed @ 1.8V pullup"
io8_166m_hslv_ft_hs_pd_1v8  "IO8_FT 166MHz HSLV high speed @ 1.8V pulldown"
io8_166m_hslv_ft_fs_1v8  "IO8_FT 166MHz HSLV fast speed @ 1.8V"
io8_166m_hslv_ft_fs_pu_1v8  "IO8_FT 166MHz HSLV fast speed @ 1.8V pullup"
io8_166m_hslv_ft_fs_pd_1v8  "IO8_FT 166MHz HSLV fast speed @ 1.8V pulldown"
io8_166m_hslv_ft_ms_1v8  "IO8_FT 166MHz HSLV med speed @ 1.8V"
io8_166m_hslv_ft_ms_pu_1v8  "IO8_FT 166MHz HSLV med speed @ 1.8V pullup"
io8_166m_hslv_ft_ms_pd_1v8  "IO8_FT 166MHz HSLV med speed @ 1.8V pulldown"
io8_166m_hslv_ft_ls_1v8  "IO8_FT 166MHz HSLV low speed @ 1.8V"
io8_166m_hslv_ft_ls_pu_1v8  "IO8_FT 166MHz HSLV low speed @ 1.8V pullup"
io8_166m_hslv_ft_ls_pd_1v8  "IO8_FT 166MHz HSLV low speed @ 1.8V pulldown"
io8_166m_hslv_ft_hs_2v5  "IO8_FT 166MHz HSLV high speed @ 2.5V"
io8_166m_hslv_ft_hs_pu_2v5  "IO8_FT 166MHz HSLV high speed @ 2.5V pullup"
io8_166m_hslv_ft_hs_pd_2v5  "IO8_FT 166MHz HSLV high speed @ 2.5V pulldown"
io8_166m_hslv_ft_fs_2v5  "IO8_FT 166MHz HSLV fast speed @ 2.5V"
io8_166m_hslv_ft_fs_pu_2v5  "IO8_FT 166MHz HSLV fast speed @ 2.5V pullup"
io8_166m_hslv_ft_fs_pd_2v5  "IO8_FT 166MHz HSLV fast speed @ 2.5V pulldown"
io8_166m_hslv_ft_ms_2v5  "IO8_FT 166MHz HSLV med speed @ 2.5V"
io8_166m_hslv_ft_ms_pu_2v5  "IO8_FT 166MHz HSLV med speed @ 2.5V pullup"
io8_166m_hslv_ft_ms_pd_2v5  "IO8_FT 166MHz HSLV med speed @ 2.5V pulldown"
io8_166m_hslv_ft_ls_2v5  "IO8_FT 166MHz HSLV low speed @ 2.5V"
io8_166m_hslv_ft_ls_pu_2v5  "IO8_FT 166MHz HSLV low speed @ 2.5V pullup"
io8_166m_hslv_ft_ls_pd_2v5  "IO8_FT 166MHz HSLV low speed @ 2.5V pulldown"
[Model Selector] io8_166m_hslv_i2c_ft
io8_166m_ft_hs_1v2  "IO8_FT 166MHz high speed @ 1.2V"
io8_166m_ft_hs_pu_1v2  "IO8_FT 166MHz high speed @ 1.2V pullup"
io8_166m_ft_hs_pd_1v2  "IO8_FT 166MHz high speed @ 1.2V pulldown"
io8_166m_ft_fs_1v2  "IO8_FT 166MHz fast speed @ 1.2V"
io8_166m_ft_fs_pu_1v2  "IO8_FT 166MHz fast speed @ 1.2V pullup"
io8_166m_ft_fs_pd_1v2  "IO8_FT 166MHz fast speed @ 1.2V pulldown"
io8_166m_ft_ms_1v2  "IO8_FT 166MHz med speed @ 1.2V"
io8_166m_ft_ms_pu_1v2  "IO8_FT 166MHz med speed @ 1.2V pullup"
io8_166m_ft_ms_pd_1v2  "IO8_FT 166MHz med speed @ 1.2V pulldown"
io8_166m_ft_ls_1v2  "IO8_FT 166MHz low speed @ 1.2V"
io8_166m_ft_ls_pu_1v2  "IO8_FT 166MHz low speed @ 1.2V pullup"
io8_166m_ft_ls_pd_1v2  "IO8_FT 166MHz low speed @ 1.2V pulldown"
io8_166m_ft_hs_1v8  "IO8_FT 166MHz high speed @ 1.8V"
io8_166m_ft_hs_pu_1v8  "IO8_FT 166MHz high speed @ 1.8V pullup"
io8_166m_ft_hs_pd_1v8  "IO8_FT 166MHz high speed @ 1.8V pulldown"
io8_166m_ft_fs_1v8  "IO8_FT 166MHz fast speed @ 1.8V"
io8_166m_ft_fs_pu_1v8  "IO8_FT 166MHz fast speed @ 1.8V pullup"
io8_166m_ft_fs_pd_1v8  "IO8_FT 166MHz fast speed @ 1.8V pulldown"
io8_166m_ft_ms_1v8  "IO8_FT 166MHz med speed @ 1.8V"
io8_166m_ft_ms_pu_1v8  "IO8_FT 166MHz med speed @ 1.8V pullup"
io8_166m_ft_ms_pd_1v8  "IO8_FT 166MHz med speed @ 1.8V pulldown"
io8_166m_ft_ls_1v8  "IO8_FT 166MHz low speed @ 1.8V"
io8_166m_ft_ls_pu_1v8  "IO8_FT 166MHz low speed @ 1.8V pullup"
io8_166m_ft_ls_pd_1v8  "IO8_FT 166MHz low speed @ 1.8V pulldown"
io8_166m_ft_hs_3v3  "IO8_FT 166MHz high speed @ 3.3V"
io8_166m_ft_hs_pu_3v3  "IO8_FT 166MHz high speed @ 3.3V pullup"
io8_166m_ft_hs_pd_3v3  "IO8_FT 166MHz high speed @ 3.3V pulldown"
io8_166m_ft_fs_3v3  "IO8_FT 166MHz fast speed @ 3.3V"
io8_166m_ft_fs_pu_3v3  "IO8_FT 166MHz fast speed @ 3.3V pullup"
io8_166m_ft_fs_pd_3v3  "IO8_FT 166MHz fast speed @ 3.3V pulldown"
io8_166m_ft_ms_3v3  "IO8_FT 166MHz med speed @ 3.3V"
io8_166m_ft_ms_pu_3v3  "IO8_FT 166MHz med speed @ 3.3V pullup"
io8_166m_ft_ms_pd_3v3  "IO8_FT 166MHz med speed @ 3.3V pulldown"
io8_166m_ft_ls_3v3  "IO8_FT 166MHz low speed @ 3.3V"
io8_166m_ft_ls_pu_3v3  "IO8_FT 166MHz low speed @ 3.3V pullup"
io8_166m_ft_ls_pd_3v3  "IO8_FT 166MHz low speed @ 3.3V pulldown"
io8_166m_hslv_ft_hs_1v2  "IO8_FT 166MHz HSLV high speed @ 1.2V"
io8_166m_hslv_ft_hs_pu_1v2  "IO8_FT 166MHz HSLV high speed @ 1.2V pullup"
io8_166m_hslv_ft_hs_pd_1v2  "IO8_FT 166MHz HSLV high speed @ 1.2V pulldown"
io8_166m_hslv_ft_fs_1v2  "IO8_FT 166MHz HSLV fast speed @ 1.2V"
io8_166m_hslv_ft_fs_pu_1v2  "IO8_FT 166MHz HSLV fast speed @ 1.2V pullup"
io8_166m_hslv_ft_fs_pd_1v2  "IO8_FT 166MHz HSLV fast speed @ 1.2V pulldown"
io8_166m_hslv_ft_ms_1v2  "IO8_FT 166MHz HSLV med speed @ 1.2V"
io8_166m_hslv_ft_ms_pu_1v2  "IO8_FT 166MHz HSLV med speed @ 1.2V pullup"
io8_166m_hslv_ft_ms_pd_1v2  "IO8_FT 166MHz HSLV med speed @ 1.2V pulldown"
io8_166m_hslv_ft_ls_1v2  "IO8_FT 166MHz HSLV low speed @ 1.2V"
io8_166m_hslv_ft_ls_pu_1v2  "IO8_FT 166MHz HSLV low speed @ 1.2V pullup"
io8_166m_hslv_ft_ls_pd_1v2  "IO8_FT 166MHz HSLV low speed @ 1.2V pulldown"
io8_166m_hslv_ft_hs_1v8  "IO8_FT 166MHz HSLV high speed @ 1.8V"
io8_166m_hslv_ft_hs_pu_1v8  "IO8_FT 166MHz HSLV high speed @ 1.8V pullup"
io8_166m_hslv_ft_hs_pd_1v8  "IO8_FT 166MHz HSLV high speed @ 1.8V pulldown"
io8_166m_hslv_ft_fs_1v8  "IO8_FT 166MHz HSLV fast speed @ 1.8V"
io8_166m_hslv_ft_fs_pu_1v8  "IO8_FT 166MHz HSLV fast speed @ 1.8V pullup"
io8_166m_hslv_ft_fs_pd_1v8  "IO8_FT 166MHz HSLV fast speed @ 1.8V pulldown"
io8_166m_hslv_ft_ms_1v8  "IO8_FT 166MHz HSLV med speed @ 1.8V"
io8_166m_hslv_ft_ms_pu_1v8  "IO8_FT 166MHz HSLV med speed @ 1.8V pullup"
io8_166m_hslv_ft_ms_pd_1v8  "IO8_FT 166MHz HSLV med speed @ 1.8V pulldown"
io8_166m_hslv_ft_ls_1v8  "IO8_FT 166MHz HSLV low speed @ 1.8V"
io8_166m_hslv_ft_ls_pu_1v8  "IO8_FT 166MHz HSLV low speed @ 1.8V pullup"
io8_166m_hslv_ft_ls_pd_1v8  "IO8_FT 166MHz HSLV low speed @ 1.8V pulldown"
io8_166m_hslv_ft_hs_2v5  "IO8_FT 166MHz HSLV high speed @ 2.5V"
io8_166m_hslv_ft_hs_pu_2v5  "IO8_FT 166MHz HSLV high speed @ 2.5V pullup"
io8_166m_hslv_ft_hs_pd_2v5  "IO8_FT 166MHz HSLV high speed @ 2.5V pulldown"
io8_166m_hslv_ft_fs_2v5  "IO8_FT 166MHz HSLV fast speed @ 2.5V"
io8_166m_hslv_ft_fs_pu_2v5  "IO8_FT 166MHz HSLV fast speed @ 2.5V pullup"
io8_166m_hslv_ft_fs_pd_2v5  "IO8_FT 166MHz HSLV fast speed @ 2.5V pulldown"
io8_166m_hslv_ft_ms_2v5  "IO8_FT 166MHz HSLV med speed @ 2.5V"
io8_166m_hslv_ft_ms_pu_2v5  "IO8_FT 166MHz HSLV med speed @ 2.5V pullup"
io8_166m_hslv_ft_ms_pd_2v5  "IO8_FT 166MHz HSLV med speed @ 2.5V pulldown"
io8_166m_hslv_ft_ls_2v5  "IO8_FT 166MHz HSLV low speed @ 2.5V"
io8_166m_hslv_ft_ls_pu_2v5  "IO8_FT 166MHz HSLV low speed @ 2.5V pullup"
io8_166m_hslv_ft_ls_pd_2v5  "IO8_FT 166MHz HSLV low speed @ 2.5V pulldown"
io8_166m_i2c_ft_1v2  "IO8_FT 166MHz I2C @ 1.2V"
io8_166m_i2c_ft_pu_1v2  "IO8_FT 166MHz I2C @ 1.2V pullup"
io8_166m_i2c_ft_pd_1v2  "IO8_FT 166MHz I2C @ 1.2V pulldown"
io8_166m_i2c_ft_1v8  "IO8_FT 166MHz I2C @ 1.8V"
io8_166m_i2c_ft_pu_1v8  "IO8_FT 166MHz I2C @ 1.8V pullup"
io8_166m_i2c_ft_pd_1v8  "IO8_FT 166MHz I2C @ 1,8V pulldown"
io8_166m_i2c_ft_3v3  "IO8_FT 166MHz I2C @ 3.3V"
io8_166m_i2c_ft_pu_3v3  "IO8_FT 166MHz I2C HSLV @ 3.3V pullup"
io8_166m_i2c_ft_pd_3v3  "IO8_FT 166MHz I2C @ 3.3V pulldown"
[Model Selector] io8_100m_ft_v33
io8_ft_v33_hs_1v2  "IO8_FT_V33 high speed @ 1.2V"
io8_ft_v33_hs_pu_1v2  "IO8_FT_V33 high speed @ 1.2V pullup"
io8_ft_v33_hs_pd_1v2  "IO8_FT_V33 high speed @ 1.2V pulldown"
io8_ft_v33_fs_1v2  "IO8_FT_V33 fast speed @ 1.2V"
io8_ft_v33_fs_pu_1v2  "IO8_FT_V33 fast speed @ 1.2V pullup"
io8_ft_v33_fs_pd_1v2  "IO8_FT_V33 fast speed @ 1.2V pulldown"
io8_ft_v33_ms_1v2  "IO8_FT_V33 med speed @ 1.2V"
io8_ft_v33_ms_pu_1v2  "IO8_FT_V33 med speed @ 1.2V pullup"
io8_ft_v33_ms_pd_1v2  "IO8_FT_V33 med speed @ 1.2V pulldown"
io8_ft_v33_ls_1v2  "IO8_FT_V33 low speed @ 1.2V"
io8_ft_v33_ls_pu_1v2  "IO8_FT_V33 low speed @ 1.2V pullup"
io8_ft_v33_ls_pd_1v2  "IO8_FT_V33 low speed @ 1.2V pulldown"
io8_ft_v33_hs_1v8  "IO8_FT_V33 high speed @ 1.8V"
io8_ft_v33_hs_pu_1v8  "IO8_FT_V33 high speed @ 1.8V pullup"
io8_ft_v33_hs_pd_1v8  "IO8_FT_V33 high speed @ 1.8V pulldown"
io8_ft_v33_fs_1v8  "IO8_FT_V33 fast speed @ 1.8V"
io8_ft_v33_fs_pu_1v8  "IO8_FT_V33 fast speed @ 1.8V pullup"
io8_ft_v33_fs_pd_1v8  "IO8_FT_V33 fast speed @ 1.8V pulldown"
io8_ft_v33_ms_1v8  "IO8_FT_V33 med speed @ 1.8V"
io8_ft_v33_ms_pu_1v8  "IO8_FT_V33 med speed @ 1.8V pullup"
io8_ft_v33_ms_pd_1v8  "IO8_FT_V33 med speed @ 1.8V pulldown"
io8_ft_v33_ls_1v8  "IO8_FT_V33 low speed @ 1.8V"
io8_ft_v33_ls_pu_1v8  "IO8_FT_V33 low speed @ 1.8V pullup"
io8_ft_v33_ls_pd_1v8  "IO8_FT_V33 low speed @ 1.8V pulldown"
io8_ft_v33_hs_3v3  "IO8_FT_V33 high speed @ 3.3V"
io8_ft_v33_hs_pu_3v3  "IO8_FT_V33 high speed @ 3.3V pullup"
io8_ft_v33_hs_pd_3v3  "IO8_FT_V33 high speed @ 3.3V pulldown"
io8_ft_v33_fs_3v3  "IO8_FT_V33 fast speed @ 3.3V"
io8_ft_v33_fs_pu_3v3  "IO8_FT_V33 fast speed @ 3.3V pullup"
io8_ft_v33_fs_pd_3v3  "IO8_FT_V33 fast speed @ 3.3V pulldown"
io8_ft_v33_ms_3v3  "IO8_FT_V33 med speed @ 3.3V"
io8_ft_v33_ms_pu_3v3  "IO8_FT_V33 med speed @ 3.3V pullup"
io8_ft_v33_ms_pd_3v3  "IO8_FT_V33 med speed @ 3.3V pulldown"
io8_ft_v33_ls_3v3  "IO8_FT_V33 low speed @ 3.3V"
io8_ft_v33_ls_pu_3v3  "IO8_FT_V33 low speed @ 3.3V pullup"
io8_ft_v33_ls_pd_3v3  "IO8_FT_V33 low speed @ 3.3V pulldown"
[Model Selector] io8_spi_ft
io8_spi_ft_hs_1v2  "IO8_FT SPI high speed @ 1.2V"
io8_spi_ft_hs_pu_1v2  "IO8_FT SPI high speed @ 1.2V pullup"
io8_spi_ft_hs_pd_1v2  "IO8_FT SPI high speed @ 1.2V pulldown"
io8_spi_ft_fs_1v2  "IO8_FT SPI fast speed @ 1.2V"
io8_spi_ft_fs_pu_1v2  "IO8_FT SPI fast speed @ 1.2V pullup"
io8_spi_ft_fs_pd_1v2  "IO8_FT SPI fast speed @ 1.2V pulldown"
io8_spi_ft_ms_1v2  "IO8_FT SPI med speed @ 1.2V"
io8_spi_ft_ms_pu_1v2  "IO8_FT SPI med speed @ 1.2V pullup"
io8_spi_ft_ms_pd_1v2  "IO8_FT SPI med speed @ 1.2V pulldown"
io8_spi_ft_ls_1v2  "IO8_FT SPI low speed @ 1.2V"
io8_spi_ft_ls_pu_1v2  "IO8_FT SPI low speed @ 1.2V pullup"
io8_spi_ft_ls_pd_1v2  "IO8_FT SPI low speed @ 1.2V pulldown"
io8_spi_ft_hs_1v8  "IO8_FT SPI high speed @ 1.8V"
io8_spi_ft_hs_pu_1v8  "IO8_FT SPI high speed @ 1.8V pullup"
io8_spi_ft_hs_pd_1v8  "IO8_FT SPI high speed @ 1.8V pulldown"
io8_spi_ft_fs_1v8  "IO8_FT SPI fast speed @ 1.8V"
io8_spi_ft_fs_pu_1v8  "IO8_FT SPI fast speed @ 1.8V pullup"
io8_spi_ft_fs_pd_1v8  "IO8_FT SPI fast speed @ 1.8V pulldown"
io8_spi_ft_ms_1v8  "IO8_FT SPI med speed @ 1.8V"
io8_spi_ft_ms_pu_1v8  "IO8_FT SPI med speed @ 1.8V pullup"
io8_spi_ft_ms_pd_1v8  "IO8_FT SPI med speed @ 1.8V pulldown"
io8_spi_ft_ls_1v8  "IO8_FT SPI low speed @ 1.8V"
io8_spi_ft_ls_pu_1v8  "IO8_FT SPI low speed @ 1.8V pullup"
io8_spi_ft_ls_pd_1v8  "IO8_FT SPI low speed @ 1.8V pulldown"
io8_spi_ft_hs_3v3  "IO8_FT SPI high speed @ 3.3V"
io8_spi_ft_hs_pu_3v3  "IO8_FT SPI high speed @ 3.3V pullup"
io8_spi_ft_hs_pd_3v3  "IO8_FT SPI high speed @ 3.3V pulldown"
io8_spi_ft_fs_3v3  "IO8_FT SPI fast speed @ 3.3V"
io8_spi_ft_fs_pu_3v3  "IO8_FT SPI fast speed @ 3.3V pullup"
io8_spi_ft_fs_pd_3v3  "IO8_FT SPI fast speed @ 3.3V pulldown"
io8_spi_ft_ms_3v3  "IO8_FT SPI med speed @ 3.3V"
io8_spi_ft_ms_pu_3v3  "IO8_FT SPI med speed @ 1.8V pullup"
io8_spi_ft_ms_pd_3v3  "IO8_FT SPI med speed @ 3.3V pulldown"
io8_spi_ft_ls_3v3  "IO8_FT SPI low speed @ 3.3V"
io8_spi_ft_ls_pu_3v3  "IO8_FT SPI low speed @ 3.3V pullup"
io8_spi_ft_ls_pd_3v3  "IO8_FT SPI low speed @ 3.3V pulldown"
io8_spi_hslv_ft_hs_1v2  "IO8_FT SPI HSLV high speed @ 1.2V"
io8_spi_hslv_ft_hs_pu_1v2  "IO8_FT SPI HSLV high speed @ 1.2V pullup"
io8_spi_hslv_ft_hs_pd_1v2  "IO8_FT SPI HSLV high speed @ 1.2V pulldown"
io8_spi_hslv_ft_fs_1v2  "IO8_FT SPI HSLV fast speed @ 1.2V"
io8_spi_hslv_ft_fs_pu_1v2  "IO8_FT SPI HSLV fast speed @ 1.2V pullup"
io8_spi_hslv_ft_fs_pd_1v2  "IO8_FT SPI HSLV fast speed @ 1.2V pulldown"
io8_spi_hslv_ft_ms_1v2  "IO8_FT SPI HSLV med speed @ 1.2V"
io8_spi_hslv_ft_ms_pu_1v2  "IO8_FT SPI HSLV med speed @ 1.2V pullup"
io8_spi_hslv_ft_ms_pd_1v2  "IO8_FT SPI HSLV med speed @ 1.2V pulldown"
io8_spi_hslv_ft_ls_1v2  "IO8_FT SPI HSLV low speed @ 1.2V"
io8_spi_hslv_ft_ls_pu_1v2  "IO8_FT SPI HSLV low speed @ 1.2V pullup"
io8_spi_hslv_ft_ls_pd_1v2  "IO8_FT SPI HSLV low speed @ 1.2V pulldown"
io8_spi_hslv_ft_hs_1v8  "IO8_FT SPI HSLV high speed @ 1.8V"
io8_spi_hslv_ft_hs_pu_1v8  "IO8_FT SPI HSLV high speed @ 1.8V pullup"
io8_spi_hslv_ft_hs_pd_1v8  "IO8_FT SPI HSLV high speed @ 1.8V pulldown"
io8_spi_hslv_ft_fs_1v8  "IO8_FT SPI HSLV fast speed @ 1.8V"
io8_spi_hslv_ft_fs_pu_1v8  "IO8_FT SPI HSLV fast speed @ 1.8V pullup"
io8_spi_hslv_ft_fs_pd_1v8  "IO8_FT SPI HSLV fast speed @ 1.8V pulldown"
io8_spi_hslv_ft_ms_1v8  "IO8_FT SPI HSLV med speed @ 1.8V"
io8_spi_hslv_ft_ms_pu_1v8  "IO8_FT SPI HSLV med speed @ 1.8V pullup"
io8_spi_hslv_ft_ms_pd_1v8  "IO8_FT SPI HSLV med speed @ 1.8V pulldown"
io8_spi_hslv_ft_ls_1v8  "IO8_FT SPI HSLV low speed @ 1.8V"
io8_spi_hslv_ft_ls_pu_1v8  "IO8_FT SPI HSLV low speed @ 1.8V pullup"
io8_spi_hslv_ft_ls_pd_1v8  "IO8_FT SPI HSLV low speed @ 1.8V pulldown"
io8_spi_hslv_ft_hs_2v5  "IO8_FT SPI HSLV high speed @ 2.5V"
io8_spi_hslv_ft_hs_pu_2v5  "IO8_FT SPI HSLV high speed @ 2.5V pullup"
io8_spi_hslv_ft_hs_pd_2v5  "IO8_FT SPI HSLV high speed @ 2.5V pulldown"
io8_spi_hslv_ft_fs_2v5  "IO8_FT SPI HSLV fast speed @ 2.5V"
io8_spi_hslv_ft_fs_pu_2v5  "IO8_FT SPI HSLV fast speed @ 2.5V pullup"
io8_spi_hslv_ft_fs_pd_2v5  "IO8_FT SPI HSLV fast speed @ 2.5V pulldown"
io8_spi_hslv_ft_ms_2v5  "IO8_FT SPI HSLV med speed @ 2.5V"
io8_spi_hslv_ft_ms_pu_2v5  "IO8_FT SPI HSLV med speed @ 2.5V pullup"
io8_spi_hslv_ft_ms_pd_2v5  "IO8_FT SPI HSLV med speed @ 2.5V pulldown"
io8_spi_hslv_ft_ls_2v5  "IO8_FT SPI HSLV low speed @ 2.5V"
io8_spi_hslv_ft_ls_pu_2v5  "IO8_FT SPI HSLV low speed @ 2.5V pullup"
io8_spi_hslv_ft_ls_pd_2v5  "IO8_FT SPI HSLV low speed @ 2.5V pulldown"
[Define Package Model]  476-ufbga-10x10-144-smps-230223
[Manufacturer]  unknown
[OEM]  unknown
[Description]  unknown
[Number Of Pins]  125
[Pin Numbers]
| Pin Name Terminal   Net Name   Starting Node   Ending Node
F1 | DSI_CKN
F2 | DSI_CKP
E1 | DSI_D0N
E2 | DSI_D0P
G1 | DSI_D1N
G2 | DSI_D1P
J2 | NRST
H4 | PA0
K3 | PA1
L2 | PA2
M2 | PA3
L3 | PA4
K4 | PA5
M3 | PA6
L4 | PA7
D11 | PA8
E9 | PA9
B12 | PA10
C12 | PA11
C11 | PA12
C10 | PA13
B11 | PA14
C9 | PA15
J5 | PB0
M4 | PB1
H6 | PB2
D6 | PB3
A5 | PB4
B5 | PB5
A4 | PB6
C5 | PB7
B4 | PB8
A2 | PB9
K8 | PB10
L7 | PB11
M10 | PB13
L10 | PB14
M9 | PB15
K2 | PC0
K1 | PC1
G5 | PC2
L1 | PC3
G9 | PC6
F9 | PC7
D12 | PC8
F8 | PC9
B10 | PC10
C8 | PC11
A11 | PC12
E4 | PC13
C1 | PC14-OSC32_IN
D2 | PC15-OSC32_OUT
D8 | PD0
E7 | PD1
B9 | PD2
A10 | PD3
C7 | PD4
B8 | PD5
D7 | PD6
A9 | PD7
M11 | PD8
K10 | PD9
L11 | PD10
L9 | PD11
K11 | PD12
K9 | PD13
L12 | PD14
H9 | PD15
B3 | PE0
B1 | PE2
B2 | PE3
C3 | PE4
C4 | PE5
D3 | PE6
L5 | PE7
H8 | PE8
K6 | PE9
J7 | PE10
M5 | PE11
J8 | PE12
L6 | PE13
K7 | PE14
M6 | PE15
E5 | PF0
F4 | PF1
G4 | PF2
K5 | PG0
J6 | PG1
B7 | PG9
A8 | PG10
A7 | PG12
C6 | PG13
A6 | PG14
B6 | PG15
H2 | PH0-OSC_IN
J1 | PH1-OSC_OUT
A3 | PH3-BOOT0
K12 | PH9
J12 | PH10
J11 | PH11
H11 | PH12
H12 | PH13
G11 | PH14
G12 | PH15
F11 | PI0
F12 | PI1
E11 | PI2
E12 | PI3
J9 | VDD11
D4 | VDD11
C2 | VBAT
G3 | VDD11DSI
D10 | VDDUSB
E8 | VDD
J4 | VDDA
E6 | VDDIO2
M8 | VDDSMPS
E10 | VDD
E3 | VDDDSI
M7 | VLXSMPS
H3 | VREFP
A1 | VSS
J3 | VSSA
L8 | VSSSMPS
D1 | VSSDSI
|[Merged Pins]  E8
|F5  |  VDD
|G8  |  VDD
|H5  |  VDD
|H7  |  VDD
|[Merged Pins]  E10
|G10  |  VDD
|J10  |  VDD
|[Merged Pins]  A1
|A12  |  VSS
|D5  |  VSS
|D9  |  VSS
|F6  |  VSS
|F7  |  VSS
|F10  |  VSS
|G6  |  VSS
|G7  |  VSS
|H10  |  VSS
|M1  |  VSS
|M12  |  VSS
|[Merged Pins]  D1
|F3  |  VSSDSI
|H1  |  VSSDSI
[Model Data]
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[End Model Data]
[End Package Model]
| Models and submodels in the file (274): io8_100m_ft_hs_1v2 (I/O), io8_100m_ft_hs_pu_1v2 (I/O), io8_100m_ft_hs_pd_1v2 (I/O), io8_100m_ft_fs_1v2 (I/O), io8_100m_ft_fs_pu_1v2 (I/O), io8_100m_ft_fs_pd_1v2 (I/O), io8_100m_ft_ms_1v2 (I/O), io8_100m_ft_ms_pu_1v2 (I/O), io8_100m_ft_ms_pd_1v2 (I/O), io8_100m_ft_ls_1v2 (I/O), io8_100m_ft_ls_pu_1v2 (I/O), io8_100m_ft_ls_pd_1v2 (I/O), io8_100m_ft_hs_1v8 (I/O), io8_100m_ft_hs_pu_1v8 (I/O), io8_100m_ft_hs_pd_1v8 (I/O), io8_100m_ft_fs_1v8 (I/O), io8_100m_ft_fs_pu_1v8 (I/O), io8_100m_ft_fs_pd_1v8 (I/O), io8_100m_ft_ms_1v8 (I/O), io8_100m_ft_ms_pu_1v8 (I/O), io8_100m_ft_ms_pd_1v8 (I/O), io8_100m_ft_ls_1v8 (I/O), io8_100m_ft_ls_pu_1v8 (I/O), io8_100m_ft_ls_pd_1v8 (I/O), io8_100m_ft_hs_3v3 (I/O), io8_100m_ft_hs_pu_3v3 (I/O), io8_100m_ft_hs_pd_3v3 (I/O), io8_100m_ft_fs_3v3 (I/O), io8_100m_ft_fs_pu_3v3 (I/O), io8_100m_ft_fs_pd_3v3 (I/O), io8_100m_ft_ms_3v3 (I/O), io8_100m_ft_ms_pu_3v3 (I/O), io8_100m_ft_ms_pd_3v3 (I/O), io8_100m_ft_ls_3v3 (I/O), io8_100m_ft_ls_pu_3v3 (I/O), io8_100m_ft_ls_pd_3v3 (I/O), io8_100m_hslv_ft_hs_1v2 (I/O), io8_100m_hslv_ft_hs_pu_1v2 (I/O), io8_100m_hslv_ft_hs_pd_1v2 (I/O), io8_100m_hslv_ft_fs_1v2 (I/O), io8_100m_hslv_ft_fs_pu_1v2 (I/O), io8_100m_hslv_ft_fs_pd_1v2 (I/O), io8_100m_hslv_ft_ms_1v2 (I/O), io8_100m_hslv_ft_ms_pu_1v2 (I/O), io8_100m_hslv_ft_ms_pd_1v2 (I/O), io8_100m_hslv_ft_ls_1v2 (I/O), io8_100m_hslv_ft_ls_pu_1v2 (I/O), io8_100m_hslv_ft_ls_pd_1v2 (I/O), io8_100m_hslv_ft_hs_1v8 (I/O), io8_100m_hslv_ft_hs_pu_1v8 (I/O), io8_100m_hslv_ft_hs_pd_1v8 (I/O), io8_100m_hslv_ft_fs_1v8 (I/O), io8_100m_hslv_ft_fs_pu_1v8 (I/O), io8_100m_hslv_ft_fs_pd_1v8 (I/O), io8_100m_hslv_ft_ms_1v8 (I/O), io8_100m_hslv_ft_ms_pu_1v8 (I/O), io8_100m_hslv_ft_ms_pd_1v8 (I/O), io8_100m_hslv_ft_ls_1v8 (I/O), io8_100m_hslv_ft_ls_pu_1v8 (I/O), io8_100m_hslv_ft_ls_pd_1v8 (I/O), io8_100m_hslv_ft_hs_2v5 (I/O), io8_100m_hslv_ft_hs_pu_2v5 (I/O), io8_100m_hslv_ft_hs_pd_2v5 (I/O), io8_100m_hslv_ft_fs_2v5 (I/O), io8_100m_hslv_ft_fs_pu_2v5 (I/O), io8_100m_hslv_ft_fs_pd_2v5 (I/O), io8_100m_hslv_ft_ms_2v5 (I/O), io8_100m_hslv_ft_ms_pu_2v5 (I/O), io8_100m_hslv_ft_ms_pd_2v5 (I/O), io8_100m_hslv_ft_ls_2v5 (I/O), io8_100m_hslv_ft_ls_pu_2v5 (I/O), io8_100m_hslv_ft_ls_pd_2v5 (I/O), io8_166m_ft_hs_1v2 (I/O), io8_166m_ft_hs_pu_1v2 (I/O), io8_166m_ft_hs_pd_1v2 (I/O), io8_166m_ft_fs_1v2 (I/O), io8_166m_ft_fs_pu_1v2 (I/O), io8_166m_ft_fs_pd_1v2 (I/O), io8_166m_ft_ms_1v2 (I/O), io8_166m_ft_ms_pu_1v2 (I/O)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
